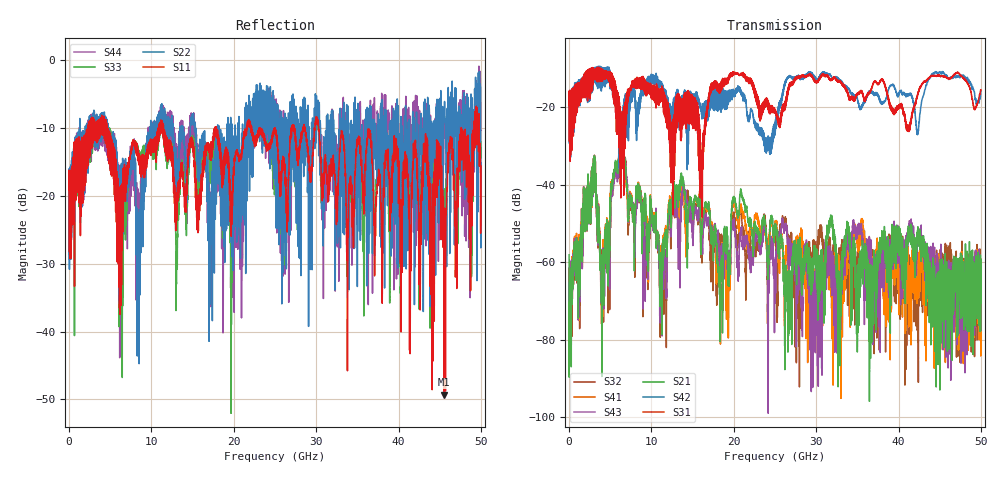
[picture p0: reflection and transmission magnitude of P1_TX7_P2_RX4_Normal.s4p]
!Keysight Technologies,N5225B,MY57041031,A.13.20.10
!Date: Friday, May 31, 2019 11:33:51
!Correction: S11(Full 4 Port(1,2,3,4))
!S12(Full 4 Port(1,2,3,4))
!S13(Full 4 Port(1,2,3,4))
!S14(Full 4 Port(1,2,3,4))
!S21(Full 4 Port(1,2,3,4))
!S22(Full 4 Port(1,2,3,4))
!S23(Full 4 Port(1,2,3,4))
!S24(Full 4 Port(1,2,3,4))
!S31(Full 4 Port(1,2,3,4))
!S32(Full 4 Port(1,2,3,4))
!S33(Full 4 Port(1,2,3,4))
!S34(Full 4 Port(1,2,3,4))
!S41(Full 4 Port(1,2,3,4))
!S42(Full 4 Port(1,2,3,4))
!S43(Full 4 Port(1,2,3,4))
!S44(Full 4 Port(1,2,3,4))
!S4P File: Measurements: <S11,S12,S13,S14>,
!<S21,S22,S23,S24>,
!<S31,S32,S33,S34>,
!<S41,S42,S43,S44>:
# Hz S  dB  R 50.0
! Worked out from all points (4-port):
!   5000 points, 10 MHz to 50 GHz, reference 50 ohm
!   strongest paths, dB at 10 MHz, 12.51 GHz, 25.01 GHz, 37.51 GHz, 50 GHz:
!     S31: -19.4, -39.2, -20.9, -14.0, -15.5
!     S42: -19.7, -27.2, -24.1, -17.0, -15.9
!     S21: -58.1, -44.4, -51.7, -58.9, -70.5
!     S43: -61.3, -44.8, -62.7, -59.5, -70.5
!     S41: -61.6, -42.8, -50.9, -55.8, -59.3
!     S32: -68.1, -45.8, -53.2, -70.7, -72.9
!   lowest |S11| = -49.3 dB at 45.52 GHz (marker M1), VSWR 1.01, Z = 49.7 + j0.0636 ohm
!   |S11| at or under -10 dB: 4.613 GHz to 10.86 GHz (6.246 GHz wide, 80.7 % of centre); 11.46 GHz to 17.73 GHz (6.278 GHz wide, 43 % of centre); 30.28 GHz to 47.61 GHz (17.33 GHz wide, 44.5 % of centre)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
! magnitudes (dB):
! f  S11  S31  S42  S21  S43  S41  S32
! 10 MHz  -19.2  -19.4  -19.7  -58.1  -61.3  -61.6  -68.1
! 6.49 GHz  -18.4  -30.5  -23.4  -29.9  -30.2  -29.8  -30.5
! 11.26 GHz  -9.2  -14.5  -14.8  -63.2  -64.4  -59.4  -66.8
! 13.78 GHz  -17.3  -18.8  -17.1  -38.4  -41.7  -40.4  -40.4
! 18.42 GHz  -13.8  -14.8  -15.7  -62.9  -59.0  -67.0  -53.0
! 45.52 GHz  -49.3  -12.0  -11.2  -66.9  -69.0  -61.2  -62.2
! 50 GHz  -15.6  -15.5  -15.9  -70.5  -70.5  -59.3  -72.9
